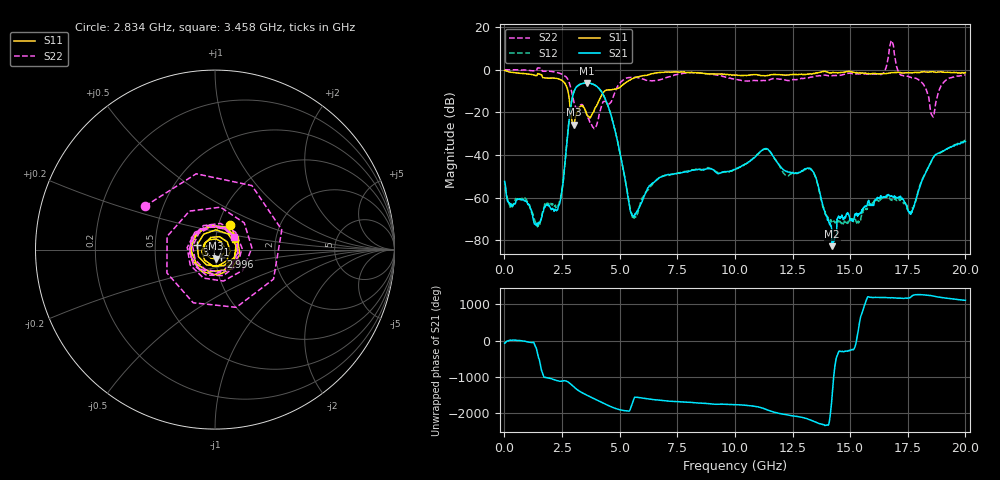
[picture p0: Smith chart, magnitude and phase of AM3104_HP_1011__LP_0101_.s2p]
!Created with skrf (http://scikit-rf.org).
# Hz S RI R 50.0
!freq ReS11 ImS11 ReS21 ImS21 ReS12 ImS12 ReS22 ImS22
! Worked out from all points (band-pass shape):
!   1601 points, 10 MHz to 20 GHz, reference 50 ohm
!   highest |S21| = -6.24 dB at 3.571 GHz (marker M1); lowest = -82.7 dB at 14.22 GHz (marker M2)
!   |S21| within 3 dB of the highest: 3.064 GHz to 4.139 GHz (1.076 GHz wide, 29.9 % of centre)
!   lowest |S11| = -25.7 dB at 3.009 GHz (marker M3), VSWR 1.11, Z = 50.3 - j5.18 ohm
!   |S11| at or under -10 dB: 2.757 GHz to 4.359 GHz (1.602 GHz wide, 45 % of centre)
!   |S22| runs from -27.7 to 13.6 dB; largest |S21 - S12| = 0.024
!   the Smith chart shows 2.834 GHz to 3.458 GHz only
!   S11 on the Smith chart (normalised r, x): 2.834 GHz: 1.13, +0.32; 2.996 GHz: 1.06, -0.09; 3.171 GHz: 0.82, +0.05; 3.458 GHz: 1.25, +0.15
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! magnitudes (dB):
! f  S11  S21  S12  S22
! 10 MHz  -0.4  -52.4  -55.3  0.0
! 1.434 GHz  -2.2  -73.2  -73.6  0.7
! 2.259 GHz  -4.1  -66.2  -64.1  -1.3
! 2.496 GHz  -5.1  -57.1  -56.6  -2.1
! 2.834 GHz  -15.8  -21.1  -21.1  -6.8
! 2.996 GHz  -25.7  -11.1  -11.1  -14.3
! 3.009 GHz  -25.7  -10.7  -10.7  -14.8
! 3.171 GHz  -19.7  -7.7  -7.7  -18.0
! 3.346 GHz  -17.0  -6.7  -6.7  -16.4
! 3.458 GHz  -17.9  -6.4  -6.4  -17.9
! 3.571 GHz  -20.7  -6.2  -6.3  -21.0
! 4.52 GHz  -9.5  -17.7  -17.8  -16.0
! 5.57 GHz  -4.2  -68.3  -68.8  -3.7
! 6.682 GHz  -1.4  -50.9  -51.0  -5.0
! 10.01 GHz  -2.7  -46.9  -46.8  -4.6
! 11.33 GHz  -2.9  -37.1  -37.3  -5.1
! 13.34 GHz  -2.1  -47.2  -47.2  -3.5
! 14.22 GHz  -1.5  -82.7  -70.8  -2.8
! 16.68 GHz  -1.6  -58.7  -59.8  7.2
! 17.65 GHz  -1.5  -67.1  -66.6  -3.7
! 18.58 GHz  -1.0  -41.8  -41.9  -21.8
! 20 GHz  -1.5  -33.7  -33.1  -2.5
